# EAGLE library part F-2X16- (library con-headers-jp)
FEMALE HEADER
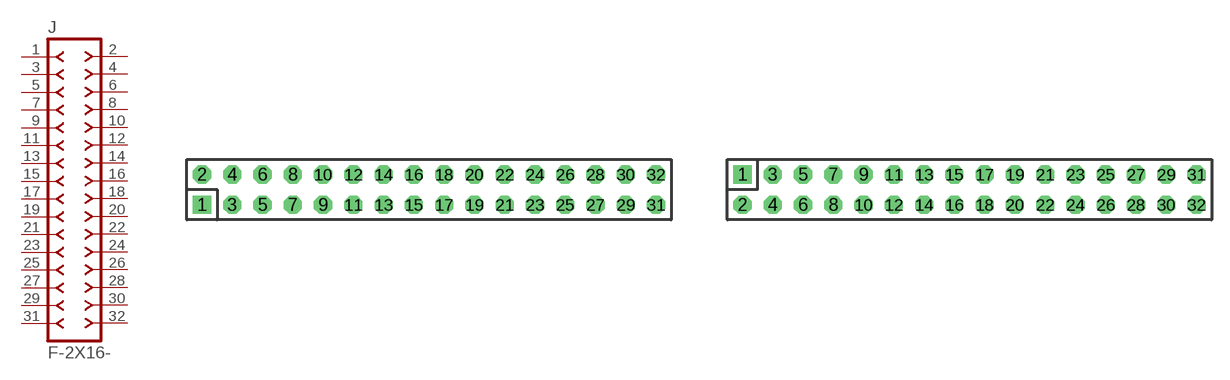
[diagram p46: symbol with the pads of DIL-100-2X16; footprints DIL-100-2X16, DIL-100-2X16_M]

Designator prefix J

## F-2X16-DIL-100  [DIL-100-2X16]
1  1  pas
2  2  pas
3  3  pas
4  4  pas
5  5  pas
6  6  pas
7  7  pas
8  8  pas
9  9  pas
10  10  pas
11  11  pas
12  12  pas
13  13  pas
14  14  pas
15  15  pas
16  16  pas
17  17  pas
18  18  pas
19  19  pas
20  20  pas
21  21  pas
22  22  pas
23  23  pas
24  24  pas
25  25  pas
26  26  pas
27  27  pas
28  28  pas
29  29  pas
30  30  pas
31  31  pas
32  32  pas

## F-2X16-DIL-100_M  [DIL-100-2X16_M]
Pads as for DIL-100-2X16

## F-2X16-DIL-2MM  [DIL-2MM-2X16]
Pads as for DIL-100-2X16

## F-2X16-DIL-2MM_M  [DIL-2MM-2X16_M]
Pads as for DIL-100-2X16

## F-2X16-71991  [71991-32]
Pads as for DIL-100-2X16

## Footprint DIL-100-2X16 (pad centres in mm)
PIN HEADER - 0.1"
drill 1.016 square: 1 -19.05,-1.27
drill 1.016 octagon: 2 -19.05,1.27; 3 -16.51,-1.27; 4 -16.51,1.27; 5 -13.97,-1.27; 6 -13.97,1.27; 7 -11.43,-1.27; 8 -11.43,1.27; 9 -8.89,-1.27; 10 -8.89,1.27; 11 -6.35,-1.27; 12 -6.35,1.27; 13 -3.81,-1.27; 14 -3.81,1.27; 15 -1.27,-1.27; 16 -1.27,1.27; 17 1.27,-1.27; 18 1.27,1.27; 19 3.81,-1.27; 20 3.81,1.27; 21 6.35,-1.27; 22 6.35,1.27; 23 8.89,-1.27; 24 8.89,1.27; 25 11.43,-1.27; 26 11.43,1.27; 27 13.97,-1.27; 28 13.97,1.27; 29 16.51,-1.27; 30 16.51,1.27; 31 19.05,-1.27; 32 19.05,1.27

## Footprint DIL-100-2X16_M (pad centres in mm)
PIN HEADER - MIRRORED 0.1"
drill 1.016 square: 1 -19.05,1.27
drill 1.016 octagon: 2 -19.05,-1.27; 3 -16.51,1.27; 4 -16.51,-1.27; 5 -13.97,1.27; 6 -13.97,-1.27; 7 -11.43,1.27; 8 -11.43,-1.27; 9 -8.89,1.27; 10 -8.89,-1.27; 11 -6.35,1.27; 12 -6.35,-1.27; 13 -3.81,1.27; 14 -3.81,-1.27; 15 -1.27,1.27; 16 -1.27,-1.27; 17 1.27,1.27; 18 1.27,-1.27; 19 3.81,1.27; 20 3.81,-1.27; 21 6.35,1.27; 22 6.35,-1.27; 23 8.89,1.27; 24 8.89,-1.27; 25 11.43,1.27; 26 11.43,-1.27; 27 13.97,1.27; 28 13.97,-1.27; 29 16.51,1.27; 30 16.51,-1.27; 31 19.05,1.27; 32 19.05,-1.27

## Footprint DIL-2MM-2X16 (pad centres in mm)
PIN HEADER - 2MM
drill 0.711 square: 1 -15,-1
drill 0.711: 2 -15,1; 3 -13,-1; 4 -13,1; 5 -11,-1; 6 -11,1; 7 -9,-1; 8 -9,1; 9 -7,-1; 10 -7,1; 11 -5,-1; 12 -5,1; 13 -3,-1; 14 -3,1; 15 -1,-1; 16 -1,1; 17 1,-1; 18 1,1; 19 3,-1; 20 3,1; 21 5,-1; 22 5,1; 23 7,-1; 24 7,1; 25 9,-1; 26 9,1; 27 11,-1; 28 11,1; 29 13,-1; 30 13,1; 31 15,-1; 32 15,1

## Footprint DIL-2MM-2X16_M (pad centres in mm)
PIN HEADER - MIRRORED 2MM
drill 0.711 square: 1 -15,1
drill 0.711: 2 -15,-1; 3 -13,1; 4 -13,-1; 5 -11,1; 6 -11,-1; 7 -9,1; 8 -9,-1; 9 -7,1; 10 -7,-1; 11 -5,1; 12 -5,-1; 13 -3,1; 14 -3,-1; 15 -1,1; 16 -1,-1; 17 1,1; 18 1,-1; 19 3,1; 20 3,-1; 21 5,1; 22 5,-1; 23 7,1; 24 7,-1; 25 9,1; 26 9,-1; 27 11,1; 28 11,-1; 29 13,1; 30 13,-1; 31 15,1; 32 15,-1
